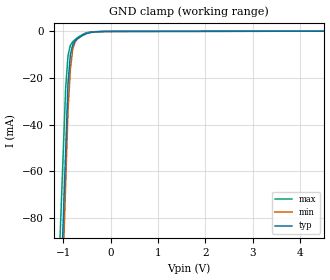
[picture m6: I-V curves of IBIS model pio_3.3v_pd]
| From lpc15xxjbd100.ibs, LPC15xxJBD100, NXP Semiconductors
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[Model] pio_3.3v_pd
Model_type Input
Vinl = 990.000mV
Vinh = 2.31000V
C_comp 598.000fF 598.000fF 598.000fF
| variable typ   min   max
[Voltage Range] 3.30000V 3.00000V 3.60000V
[POWER Clamp Reference] 3.30000V 3.00000V 3.60000V
[GND Clamp Reference] 0.00000V 0.00000V 0.00000V
[Temperature Range]   25   85   -40
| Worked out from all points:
|   GND clamp passes 1 mA (typ) near -0.52 V on its own axis
[GND Clamp]
-3.3V     -1.418A    -1.55A     -1.295A
-950mV    -51.27mA   -65.47mA   -24.26mA
-900mV    -22.19mA   -33.9mA    -10.29mA
-850mV    -9.943mA   -16.12mA   -5.882mA
-800mV    -5.683mA   -7.62mA    -4.406mA
-750mV    -4.055mA   -4.522mA   -3.521mA
-700mV    -3.054mA   -3.238mA   -2.636mA
-550mV    -1.273mA   -1.291mA   -878.5uA
-400mV    -401.9uA   -298.7uA   -198uA
-200mV    -101.1uA   -50.06uA   -18.15uA
6.6V      134.1uA    133.5uA    143.2uA
[POWER Clamp]
-3.3V     0A         0A         0A
6.6V      0A         0A         0A
